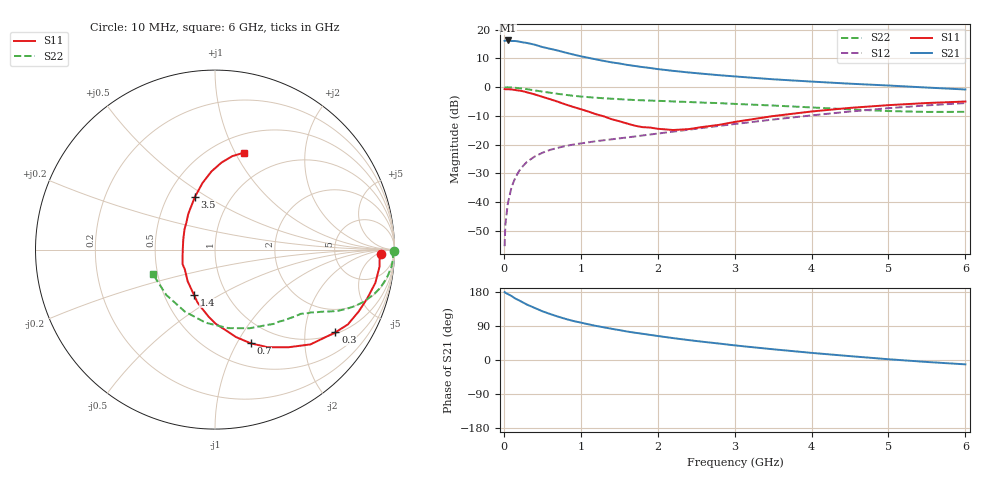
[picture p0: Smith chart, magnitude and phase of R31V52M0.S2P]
! SIEMENS Small Signal Semiconductors
! BFR181
! Si NPN RF Bipolar Junction Transistor in SOT23
! VCE = 1.5 V  IC = 2 mA
! Common Emitter S-Parameters:  May  1996
# GHz  S  MA  R  50
!  f  S11  S21  S12  S22
! GHz  MAG  ANG  MAG  ANG  MAG  ANG  MAG  ANG
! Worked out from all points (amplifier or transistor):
!   36 points, 10 MHz to 6 GHz, reference 50 ohm
!   highest |S21| = 16.3 dB at 50 MHz (marker M1)
!   |S21| within 3 dB of that: start of sweep to 617.4 MHz
!   unconditionally stable (mu >= 1): 1.541 GHz to 3.419 GHz
!   at 250 MHz: K = 0.23, MSG = 21.5 dB, |S12| = -27.4 dB
!   at 1.4 GHz: K = 0.96, MSG = 13.4 dB, |S12| = -18.2 dB
!   at 6 GHz: K = 0.88, MSG = 2.4 dB, |S12| = -5.5 dB
!   S11 on the Smith chart (normalised r, x): 10 MHz: 24, -7; 300 MHz: 1.05, -2.87; 700 MHz: 0.75, -1.14; 1.4 GHz: 0.70, -0.38; 3.5 GHz: 0.68, +0.44; 6 GHz: 0.69, +1.08
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0.01  0.9259 -1.4  6.403 179.1  0.0017 99.1  0.996 -0.6
0.02  0.9182 -2.5  6.452 177.5  0.004 93.1  0.988 -1.1
0.05  0.9218 -5.9  6.514 174.3  0.0091 86.8  0.9941 -2.8
0.1  0.9125 -11.7  6.369 168.9  0.0182 83.5  0.9878 -5.5
0.15  0.8911 -17.7  6.373 162.1  0.0267 78.9  0.9746 -8.4
0.3  0.8141 -34.5  5.891 146.3  0.05 70.4  0.9236 -15.3
0.4  0.7496 -44.8  5.509 137.5  0.0618 65.4  0.8804 -19.2
0.5  0.6804 -53.1  5.01 128.7  0.0719 61.3  0.8374 -22.2
0.6  0.6186 -61.6  4.668 121.5  0.0808 58.6  0.8014 -24.4
0.7  0.559 -69.1  4.352 114.7  0.0878 56.2  0.766 -26.4
0.8  0.5012 -76.5  4.008 108.6  0.0942 54.5  0.7358 -27.9
0.9  0.454 -82.3  3.712 103.1  0.1 53.2  0.709 -29.1
1.1  0.3759 -95.4  3.247 94.2  0.1096 52.4  0.6704 -31.3
1.2  0.3374 -102.1  3.046 89.9  0.1146 51.8  0.6549 -32.3
1.4  0.2773 -115.1  2.708 82.4  0.1234 52.1  0.6293 -34.2
1.7  0.2138 -138.7  2.345 72.1  0.1382 53.2  0.5972 -36.8
2.2  0.1795 179.1  1.925 57.8  0.1679 54.5  0.5643 -42.7
2.8  0.2209 135.9  1.616 43.4  0.2116 54.4  0.5276 -51.7
3.5  0.3137 111.0  1.372 28.3  0.273 51.8  0.4788 -66.2
4.5  0.436 92.6  1.15 10.2  0.3762 43.3  0.4106 -97.3
5.5  0.5297 79.5  0.985 -5.2  0.482 30.7  0.3708 -137.1
6  0.5629 73.5  0.912 -11.5  0.5287 23.4  0.3717 -158.2
